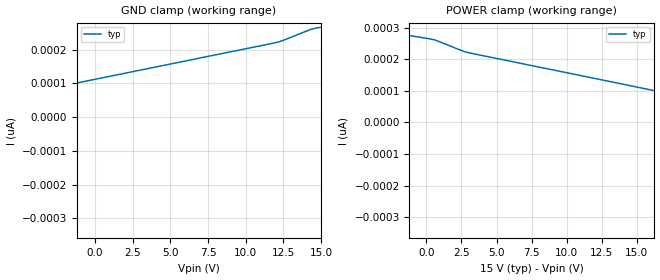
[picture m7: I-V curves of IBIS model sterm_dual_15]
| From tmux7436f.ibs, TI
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| sterm_dual_15
[Model]   sterm_dual_15
Model_type   Terminator
|   typ   min   max
C_comp   4.014581e-12   NA   NA
[Voltage Range]   15   NA   NA
[Temperature Range]   27   NA   NA
[Power Clamp Reference]   15   NA   NA
[GND Clamp Reference]   0   NA   NA
[GND Clamp]
|   Voltage   I(typ)   I(min)   I(max)
-20V      -63.89uA   NA         NA
-15.05V   -71.99nA   NA         NA
-14.7V    -23.81pA   NA         NA
11.82V    218.8pA    NA         NA
12.53V    227.9pA    NA         NA
14.29V    259.2pA    NA         NA
15V       266.1pA    NA         NA
[POWER Clamp]
|   Voltage   I(typ)   I(min)   I(max)
-5V       301.5pA    NA         NA
303mV     263.9pA    NA         NA
3.131V    219.3pA    NA         NA
29.65V    -23.26pA   NA         NA
30V       -10.3nA    NA         NA
